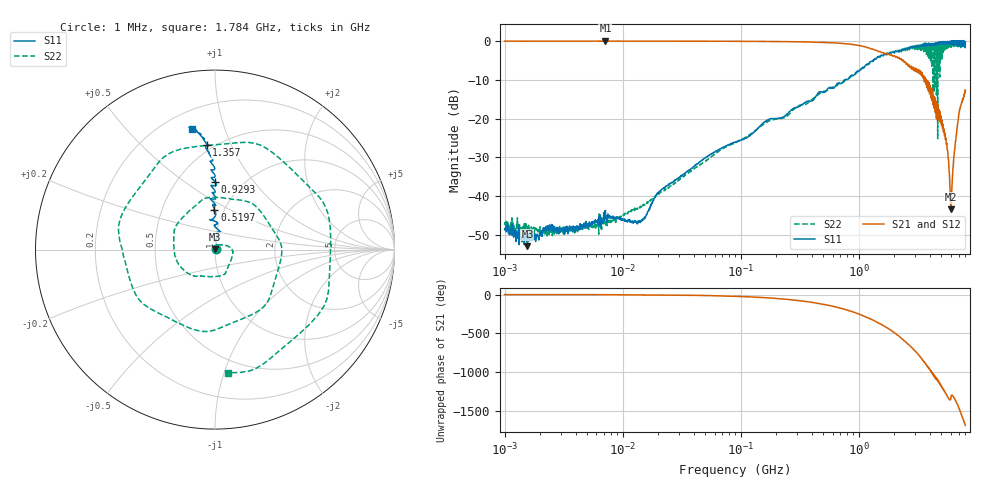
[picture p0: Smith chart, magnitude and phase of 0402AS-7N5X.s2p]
!s-Parameter Generated by FASTRON Sdn. Bhd.
!FASTRON P/N : 0402AS-7N5X
!Keysight Technologies: E5071C_MY46733604_B.14.02
!Date: Mon Dec 01 10:26:40 2025
!Version  :Rev00  Mon Dec 01 10:26:40 2025
!Data & Calibration Information:
!Freq  S11:SOLT2(ON)  S21:SOLT2(ON)  S12:SOLT2(ON)  S22:SOLT2(ON)
!PortZ  Port1:50+j0  Port2:50+j0
!When reading reference impedance value at option line is always used.
! Remarks : This data is being provided solely for informational purposes.
# Hz S dB R 50
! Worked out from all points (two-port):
!   1601 points, 1 MHz to 8 GHz, reference 50 ohm
!   highest |S21| = 0.04 dB at 7.138 MHz (marker M1); lowest = -43.4 dB at 6.034 GHz (marker M2)
!   |S21| within 3 dB of the highest: start of sweep to 1.552 GHz
!   lowest |S11| = -52.9 dB at 1.559 MHz (marker M3), VSWR 1.00, Z = 50.2 + j0.101 ohm
!   |S11| at or under -10 dB: start of sweep to 756.2 MHz
!   |S22| runs from -50.6 to -0.1 dB; largest |S21 - S12| = 0.017
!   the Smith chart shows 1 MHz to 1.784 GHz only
!   S11 on the Smith chart (normalised r, x): 1 MHz: 1.01, +0.00; 519.7 MHz: 0.90, +0.42; 929.3 MHz: 0.75, +0.66; 1.357 GHz: 0.46, +0.81; 1.784 GHz: 0.31, +0.78
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1000000  -48.60 26.1  -0.04 -0.2  -0.03 -0.3  -47.20 13.1
1559194  -52.90 26.4  -0.04 -0.4  -0.03 -0.4  -47.40 -1.4
4479405  -47.90 37.8  -0.04 -1.2  -0.02 -1.2  -47.80 39.6
7138274  -43.70 34.6  0.04 -2.0  0.02 -1.9  -45.20 39.2
2.00676e7  -39.00 52.2  -0.05 -5.2  -0.05 -5.2  -39.50 67.8
8.994653e7  -26.10 88.2  -0.08 -23.0  -0.08 -23.0  -26.20 30.3
4.006501e8  -15.40 96.7  -0.28 -101.0  -0.27 -101.0  -15.10 -123.0
5.196823e8  -13.10 90.9  -0.40 -131.0  -0.40 -131.0  -12.90 -175.0
9.292726e8  -8.42 90.2  -0.96 126.0  -0.96 126.0  -8.65 -18.7
1.357283e9  -4.69 94.6  -2.32 19.6  -2.33 19.5  -4.71 122.0
1.589302e9  -3.77 97.2  -2.99 -34.8  -2.99 -34.9  -3.70 10.4
1.784248e9  -3.30 101.0  -3.42 -80.7  -3.43 -80.8  -3.23 -84.2
1.7949e9  -3.26 101.0  -3.39 -83.5  -3.40 -83.6  -3.35 -90.7
2.157084e9  -2.65 106.0  -4.40 -170.0  -4.40 -171.0  -2.43 92.7
2.516241e9  -1.85 113.0  -5.94 100.0  -5.92 100.0  -1.96 -95.8
2.883048e9  -1.58 121.0  -6.87 16.0  -6.85 15.8  -2.14 86.3
3.244011e9  -1.47 127.0  -7.63 -65.9  -7.60 -66.2  -1.75 -78.2
3.588581e9  -0.85 140.0  -10.50 -155.0  -10.50 -155.0  -1.02 82.3
3.95342e9  -0.87 141.0  -12.10 113.0  -12.10 112.0  -4.49 -108.0
4.324643e9  -1.05 148.0  -14.20 21.3  -14.20 20.7  -5.94 129.0
6.033702e9  0.03 -161.0  -43.40 109.0  -43.50 108.0  -1.64 18.9
8e9  -0.17 -96.9  -12.80 107.0  -12.80 107.0  -1.60 146.0
